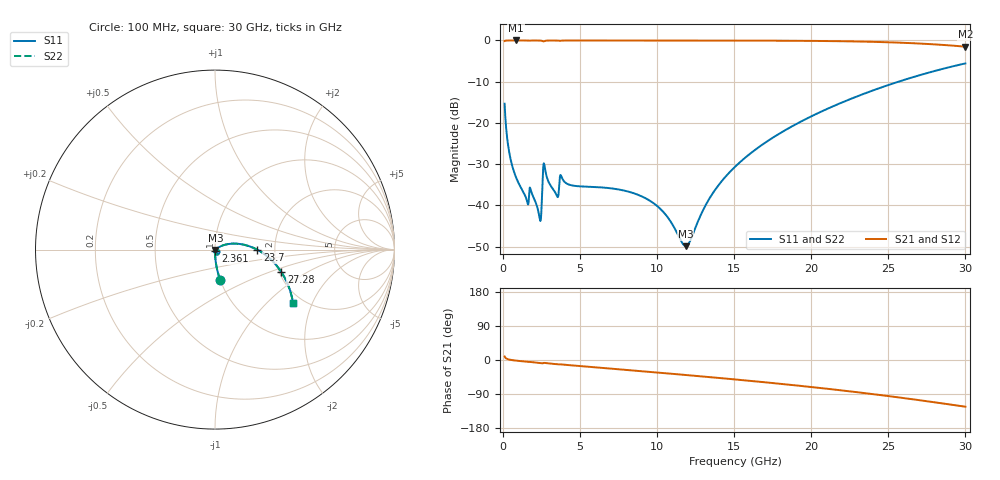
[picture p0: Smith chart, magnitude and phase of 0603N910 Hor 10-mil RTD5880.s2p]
# GHz S MA R 50
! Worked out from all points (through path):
!   3201 points, 100 MHz to 30 GHz, reference 50 ohm
!   highest |S21| = -0.01 dB at 838.2 MHz (marker M1); lowest = -1.5 dB at 30 GHz (marker M2)
!   group delay of S21, straight-line fit = 11.2 ps
!   lowest |S11| = -49.9 dB at 11.85 GHz (marker M3), VSWR 1.01, Z = 50.2 - j0.213 ohm
!   |S11| at or under -10 dB: start of sweep to 25.67 GHz
!   |S22| runs from -49.9 to -5.6 dB; largest |S21 - S12| = 0
!   S11 on the Smith chart (normalised r, x): 100 MHz: 1.00, -0.35; 2.361 GHz: 1.01, -0.01; 23.7 GHz: 1.62, -0.00; 27.28 GHz: 2.05, -0.61; 30 GHz: 1.77, -1.46
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0.1  0.1707 -80.4  0.985 9.5  0.985 9.5  0.1707 -80.4
0.4176875  0.04209 -88.3  0.9986 1.0  0.9986 1.0  0.04209 -88.3
0.8381563  0.02191 -89.6  0.999 -1.6  0.999 -1.6  0.02191 -89.6
1.52025  0.01181 -86.5  0.9983 -4.5  0.9983 -4.5  0.01181 -86.5
1.856625  0.01417 -85.8  0.9975 -5.5  0.9975 -5.5  0.01417 -85.8
2.361188  0.007143 -68.8  0.9965 -7.7  0.9965 -7.7  0.007143 -68.8
2.445281  0.006662 -37.2  0.9941 -8.2  0.9941 -8.2  0.006662 -37.2
2.6415  0.03223 -47.2  0.9748 -7.8  0.9748 -7.8  0.03223 -47.2
2.71625  0.02826 -72.6  0.9876 -7.8  0.9876 -7.8  0.02826 -72.6
3.454406  0.01348 -86.5  0.9965 -11.0  0.9965 -11.0  0.01348 -86.5
3.809469  0.02186 -88.1  0.9946 -11.8  0.9946 -11.8  0.02186 -88.1
5.089563  0.01694 -99.4  0.9978 -16.3  0.9978 -16.3  0.01694 -99.4
8.116938  0.01468 -106.8  0.9973 -26.6  0.9973 -26.6  0.01468 -106.8
10.06978  0.009548 -106.0  0.997 -33.3  0.997 -33.3  0.009548 -106.0
11.85444  0.003195 -41.5  0.9966 -39.5  0.9966 -39.5  0.003195 -41.5
13.47091  0.01279 28.5  0.9962 -45.4  0.9962 -45.4  0.01279 28.5
15.05  0.0293 31.0  0.9955 -51.3  0.9955 -51.3  0.0293 31.0
20.03956  0.121 15.9  0.987 -71.5  0.987 -71.5  0.121 15.9
23.70231  0.2361 -0.2  0.9646 -88.5  0.9646 -88.5  0.2361 -0.2
25.01978  0.2885 -6.7  0.9497 -95.3  0.9497 -95.3  0.2885 -6.7
27.28097  0.3906 -18.8  0.9117 -107.5  0.9117 -107.5  0.3906 -18.8
30  0.5265 -34.4  0.84 -123.3  0.84 -123.3  0.5265 -34.4
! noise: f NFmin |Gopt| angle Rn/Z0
0.1  0.0002735  0.9131  0.3825  0.0006932
3.417  0.004745  0.8363  11.65  0.006066
6.743  0.005753  0.7489  22.88  0.004436
10.06  0.007836  0.7321  33.8  0.005351
13.39  0.009979  0.7268  44.38  0.006251
16.7  0.01227  0.7291  54.5  0.007169
20.03  0.01481  0.737  64.18  0.008158
23.35  0.01773  0.7494  73.36  0.009268
26.67  0.02119  0.7653  82.11  0.01058
30  0.0254  0.7842  90.43  0.01218
